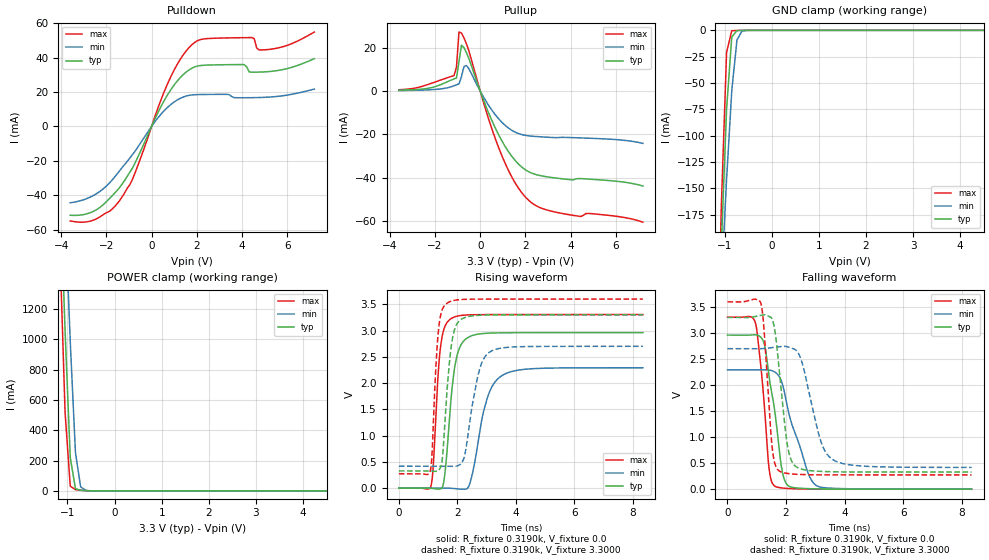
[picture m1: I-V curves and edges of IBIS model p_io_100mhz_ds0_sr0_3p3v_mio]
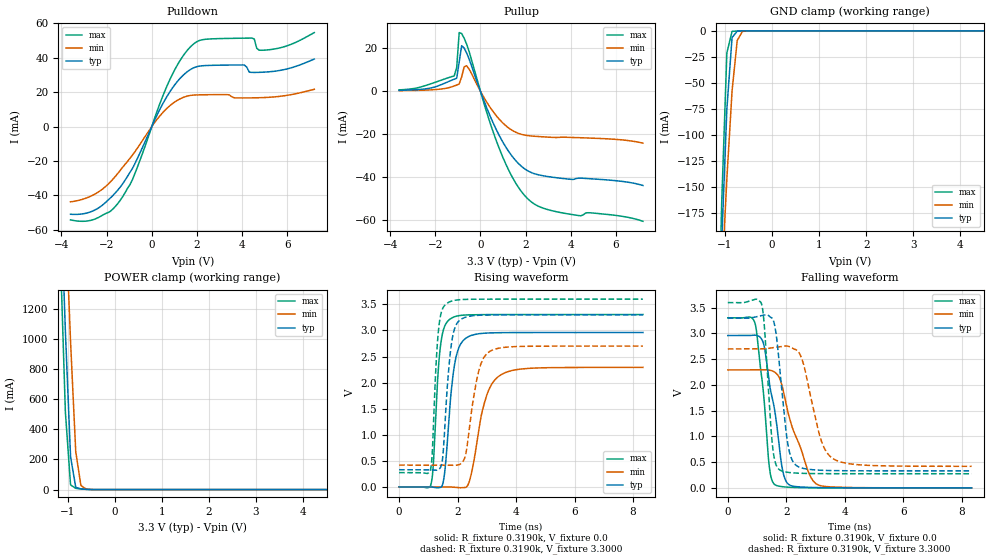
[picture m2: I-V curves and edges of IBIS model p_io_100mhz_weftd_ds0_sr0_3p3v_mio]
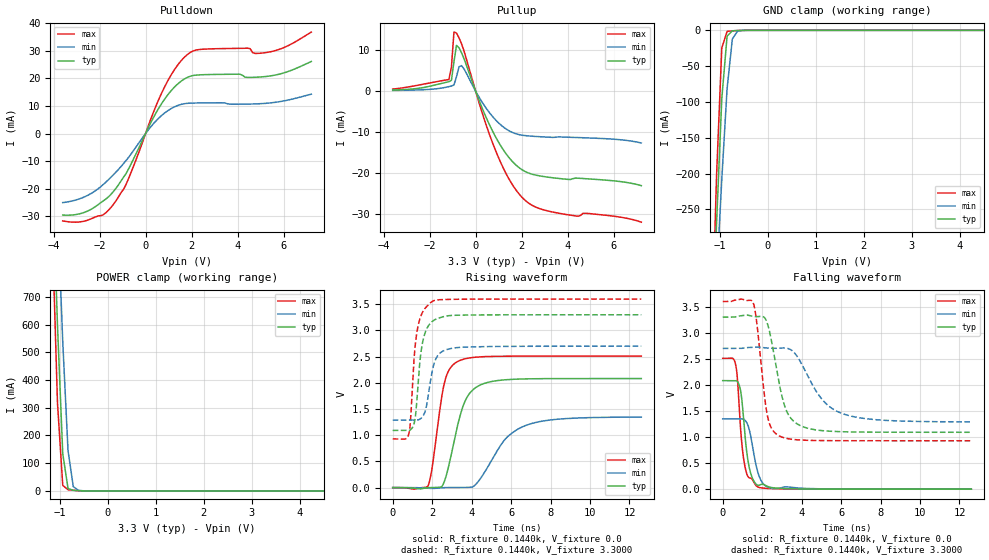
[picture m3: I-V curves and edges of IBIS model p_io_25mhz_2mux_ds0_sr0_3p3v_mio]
| IBIS file was generated by Viper version: 2025.12.22
[IBIS Ver]   6.0
[Comment Char]   |_char
[File Name]   c15x_c05x_24qfn.ibs
[File Rev]   1.0
[Date]   Fri Mar 13 19:24:16 2026
[Source]   NXP Viper 2025.12.22
[Notes]
[Disclaimer] IMPORTANT NOTICE
  This information is provided on an AS IS basis and without warranty.
  IN NO EVENT SHALL NXP BE LIABLE FOR INCIDENTAL OR CONSEQUENTIAL
  DAMAGES ARISING FROM USE OF THIS INFORMATION. THIS DISCLAIMER OF
  WARRANTY EXTENDS TO THE USER OF THE INFORMATION, AND TO THEIR CUSTOMERS
  OR USERS OF PRODUCTS  AND IS IN LIEU OF ALL WARRANTIES WHETHER EXPRESS,
  IMPLIED, OR STATUTORY, INCLUDING IMPLIED WARRANTIES OF MERCHANTABILITY
  OR FITNESS FOR PARTICULAR PURPOSE.
  NXP does not represent or warrant that the information furnished
  hereunder is free of infringement of any third party patents,
  copyrights, trade secrets, or other intellectual property rights.
  NXP does not represent or warrant that the information is free of
  defect, or that it meets any particular standard, requirements or need
  of the user of the infomation or their customers.
  NXP reserves the right to change the information in this file
  without notice.
   http://www.nxp.com
[Copyright]   (C) Copyright NXP 2004 - 2026, All Rights Reserved.
|   C15x_C05x_24QFN
[Component]   C15x_C05x_24QFN
[Manufacturer]   NXP
[Package]
| variable   typ   min   max
R_pkg   0.13896   0.12132   0.18535
L_pkg   1.804e-09   1.361e-09   2.436e-09
C_pkg   9.908e-14   8.894e-14   1.257e-13
[Pin] signal_name   model_name   R_pin   L_pin   C_pin
1   P1_9   a_ip_io_3v_3p3v   0.13781   1.901e-09 9.517e-14
2   P1_29   a_ip_io_3v_3p3v   0.12423   1.605e-09 9.039e-14
3   P1_30   a_ip_io_3v_3p3v   0.12132   1.528e-09 9.059e-14
4   P1_31   a_ip_io_3v_3p3v   0.13072   1.361e-09 1.032e-13
5   VDD   POWER   NA   NA   NA
6   P2_2   a_ip_io_3v_3p3v   0.14812   1.699e-09 1.013e-13
7   P2_3   a_ip_io_3v_3p3v   0.13439   1.749e-09 9.377e-14
8   P2_7   a_ip_io_3v_3p3v   0.12467   1.656e-09 9.088e-14
9   P2_12   a_ip_io_3v_3p3v   0.1273   1.509e-09 9.647e-14
10   P2_13   a_ip_io_3v_3p3v   0.13519   1.740e-09 1.000e-13
11   P2_16   a_ip_io_3v_3p3v   0.15539   1.988e-09 1.160e-13
12   P2_17   a_ip_io_3v_3p3v   0.18535   2.436e-09 1.257e-13
13   P3_29   a_ip_io_3v_3p3v   0.16284   2.122e-09 1.068e-13
14   P3_11   a_ip_io_3v_3p3v   0.14778   1.938e-09 1.010e-13
15   P3_10   a_ip_io_3v_3p3v   0.13217   1.797e-09 9.404e-14
16   P3_9   a_ip_io_3v_3p3v   0.12395   1.693e-09 9.041e-14
17   P3_8   a_ip_io_3v_3p3v   0.13055   1.797e-09 9.541e-14
18   P3_1   a_ip_io_3v_3p3v   0.15092   2.075e-09 1.056e-13
19   P3_0   a_ip_io_3v_3p3v   0.15252   1.996e-09 1.057e-13
20   P0_0   a_ip_io_3v_3p3v   0.12722   1.665e-09 9.034e-14
21   P0_1   a_ip_io_3v_3p3v   0.12378   1.709e-09 8.894e-14
22   P0_2   a_ip_io_3v_3p3v   0.13159   1.755e-09 9.620e-14
23   P0_3   a_ip_io_3v_3p3v   0.15143   1.961e-09 1.051e-13
24   P1_8   a_ip_io_3v_3p3v   0.13691   1.806e-09 9.582e-14
25   VSS   GND   NA   NA   NA
[Pin Mapping]   pulldown_ref   pullup_ref
1   VSS   VDD
2   VSS   VDD
3   VSS   VDD
4   VSS   VDD
5   NC   VDD
6   VSS   VDD
7   VSS   VDD
8   VSS   VDD
9   VSS   VDD
10   VSS   VDD
11   VSS   VDD
12   VSS   VDD
13   VSS   VDD
14   VSS   VDD
15   VSS   VDD
16   VSS   VDD
17   VSS   VDD
18   VSS   VDD
19   VSS   VDD
20   VSS   VDD
21   VSS   VDD
22   VSS   VDD
23   VSS   VDD
24   VSS   VDD
25   VSS   NC
|*   Model Selector   *
[Model Selector] a_ip_io_3v_3p3v
p_io_25mhz_ds0_sr0_3p3v_mio   dse=0 sre=0 25mhz
p_io_25mhz_ds0_sr1_3p3v_mio   dse=0 sre=1 25mhz
p_io_25mhz_ds1_sr0_3p3v_mio   dse=1 sre=0 25mhz
p_io_25mhz_ds1_sr1_3p3v_mio   dse=1 sre=1 25mhz
p_io_25mhz_r40_ds0_sr0_3p3v_mio   dse=0 sre=0 25mhz_r40
p_io_25mhz_r40_ds0_sr1_3p3v_mio   dse=0 sre=1 25mhz_r40
p_io_25mhz_r40_ds1_sr0_3p3v_mio   dse=1 sre=0 25mhz_r40
p_io_25mhz_r40_ds1_sr1_3p3v_mio   dse=1 sre=1 25mhz_r40
p_io_50mhz_ds0_sr0_3p3v_mio   dse=0 sre=0 50mhz
p_io_50mhz_ds0_sr1_3p3v_mio   dse=0 sre=1 50mhz
p_io_50mhz_ds1_sr0_3p3v_mio   dse=1 sre=0 50mhz
p_io_50mhz_ds1_sr1_3p3v_mio   dse=1 sre=1 50mhz
p_io_25mhz_cap_ds0_sr0_3p3v_mio   dse=0 sre=0 25mhz_cap
p_io_25mhz_cap_ds0_sr1_3p3v_mio   dse=0 sre=1 25mhz_cap
p_io_25mhz_cap_ds1_sr0_3p3v_mio   dse=1 sre=0 25mhz_cap
p_io_25mhz_cap_ds1_sr1_3p3v_mio   dse=1 sre=1 25mhz_cap
p_io_25mhz_2mux_ds0_sr0_3p3v_mio   dse=0 sre=0 25mhz_2mux
p_io_25mhz_2mux_ds0_sr1_3p3v_mio   dse=0 sre=1 25mhz_2mux
p_io_25mhz_2mux_ds1_sr0_3p3v_mio   dse=1 sre=0 25mhz_2mux
p_io_25mhz_2mux_ds1_sr1_3p3v_mio   dse=1 sre=1 25mhz_2mux
p_io_100mhz_ds0_sr0_3p3v_mio   dse=0 sre=0 100mhz
p_io_100mhz_ds0_sr1_3p3v_mio   dse=0 sre=1 100mhz
p_io_100mhz_ds1_sr0_3p3v_mio   dse=1 sre=0 100mhz
p_io_100mhz_ds1_sr1_3p3v_mio   dse=1 sre=1 100mhz
p_io_100mhz_weftd_ds0_sr0_3p3v_mio   dse=0 sre=0 100mhz
p_io_100mhz_weftd_ds0_sr1_3p3v_mio   dse=0 sre=1 100mhz
p_io_100mhz_weftd_ds1_sr0_3p3v_mio   dse=1 sre=0 100mhz
p_io_100mhz_weftd_ds1_sr1_3p3v_mio   dse=1 sre=1 100mhz
p_io_i2c_ds00_ds10_sr0_3p3v_mio   dse0=0 dse1=0 sre=0 i2c
p_io_i2c_ds00_ds10_sr1_3p3v_mio   dse0=0 dse1=0 sre=1 i2c
p_io_i2c_ds00_ds11_sr0_3p3v_mio   dse0=0 dse1=1 sre=0 i2c
p_io_i2c_ds00_ds11_sr1_3p3v_mio   dse0=0 dse1=1 sre=1 i2c
p_io_i2c_ds01_ds10_sr0_3p3v_mio   dse0=1 dse1=0 sre=0 i2c
p_io_i2c_ds01_ds10_sr1_3p3v_mio   dse0=1 dse1=0 sre=1 i2c
p_io_i2c_ds01_ds11_sr0_3p3v_mio   dse0=1 dse1=1 sre=0 i2c
p_io_i2c_ds01_ds11_sr1_3p3v_mio   dse0=1 dse1=1 sre=1 i2c
p_io_i2c_i2c1_3p3v_mio   ipp_i2c_lv=1 i2c
p_io_i2cfmp_ds00_ds10_sr0_3p3v_mio   dse0=0 dse1=0 sre=0 i2cfmp
p_io_i2cfmp_ds00_ds10_sr1_3p3v_mio   dse0=0 dse1=0 sre=1 i2cfmp
p_io_i2cfmp_ds00_ds11_sr0_3p3v_mio   dse0=0 dse1=1 sre=0 i2cfmp
p_io_i2cfmp_ds00_ds11_sr1_3p3v_mio   dse0=0 dse1=1 sre=1 i2cfmp
p_io_i2cfmp_ds01_ds10_sr0_3p3v_mio   dse0=1 dse1=0 sre=0 i2cfmp
p_io_i2cfmp_ds01_ds10_sr1_3p3v_mio   dse0=1 dse1=0 sre=1 i2cfmp
p_io_i2cfmp_ds01_ds11_sr0_3p3v_mio   dse0=1 dse1=1 sre=0 i2cfmp
p_io_i2cfmp_ds01_ds11_sr1_3p3v_mio   dse0=1 dse1=1 sre=1 i2cfmp
p_io_i2cfmp_i2c1_3p3v_mio   ipp_i2c_lv=1 i2cfmp
p_io_rst_3p3v_mio   rst
p_io_rst_rx1p8v_3p3v_mio   rst
p_io_aon_3p3v_mio   rst
| End [Component] C15x_C05x_24QFN
| Models and submodels in the file (49): p_io_100mhz_ds0_sr0_3p3v_mio (I/O), p_io_100mhz_ds0_sr1_3p3v_mio (I/O), p_io_100mhz_ds1_sr0_3p3v_mio (I/O), p_io_100mhz_ds1_sr1_3p3v_mio (I/O), p_io_100mhz_weftd_ds0_sr0_3p3v_mio (I/O), p_io_100mhz_weftd_ds0_sr1_3p3v_mio (I/O), p_io_100mhz_weftd_ds1_sr0_3p3v_mio (I/O), p_io_100mhz_weftd_ds1_sr1_3p3v_mio (I/O), p_io_25mhz_2mux_ds0_sr0_3p3v_mio (I/O), p_io_25mhz_2mux_ds0_sr1_3p3v_mio (I/O), p_io_25mhz_2mux_ds1_sr0_3p3v_mio (I/O), p_io_25mhz_2mux_ds1_sr1_3p3v_mio (I/O), p_io_25mhz_cap_ds0_sr0_3p3v_mio (I/O), p_io_25mhz_cap_ds0_sr1_3p3v_mio (I/O), p_io_25mhz_cap_ds1_sr0_3p3v_mio (I/O), p_io_25mhz_cap_ds1_sr1_3p3v_mio (I/O), p_io_25mhz_ds0_sr0_3p3v_mio (I/O), p_io_25mhz_ds0_sr1_3p3v_mio (I/O), p_io_25mhz_ds1_sr0_3p3v_mio (I/O), p_io_25mhz_ds1_sr1_3p3v_mio (I/O), p_io_25mhz_r40_ds0_sr0_3p3v_mio (I/O), p_io_25mhz_r40_ds0_sr1_3p3v_mio (I/O), p_io_25mhz_r40_ds1_sr0_3p3v_mio (I/O), p_io_25mhz_r40_ds1_sr1_3p3v_mio (I/O), p_io_50mhz_ds0_sr0_3p3v_mio (I/O), p_io_50mhz_ds0_sr1_3p3v_mio (I/O), p_io_50mhz_ds1_sr0_3p3v_mio (I/O), p_io_50mhz_ds1_sr1_3p3v_mio (I/O), p_io_aon_3p3v_mio (I/O), p_io_i2c_ds00_ds10_sr0_3p3v_mio (I/O), p_io_i2c_ds00_ds10_sr1_3p3v_mio (I/O), p_io_i2c_ds00_ds11_sr0_3p3v_mio (I/O), p_io_i2c_ds00_ds11_sr1_3p3v_mio (I/O), p_io_i2c_ds01_ds10_sr0_3p3v_mio (I/O), p_io_i2c_ds01_ds10_sr1_3p3v_mio (I/O), p_io_i2c_ds01_ds11_sr0_3p3v_mio (I/O), p_io_i2c_ds01_ds11_sr1_3p3v_mio (I/O), p_io_i2c_i2c1_3p3v_mio (I/O), p_io_i2cfmp_ds00_ds10_sr0_3p3v_mio (I/O), p_io_i2cfmp_ds00_ds10_sr1_3p3v_mio (I/O), p_io_i2cfmp_ds00_ds11_sr0_3p3v_mio (I/O), p_io_i2cfmp_ds00_ds11_sr1_3p3v_mio (I/O), p_io_i2cfmp_ds01_ds10_sr0_3p3v_mio (I/O), p_io_i2cfmp_ds01_ds10_sr1_3p3v_mio (I/O), p_io_i2cfmp_ds01_ds11_sr0_3p3v_mio (I/O), p_io_i2cfmp_ds01_ds11_sr1_3p3v_mio (I/O), p_io_i2cfmp_i2c1_3p3v_mio (I/O), p_io_rst_3p3v_mio (I/O), p_io_rst_rx1p8v_3p3v_mio (I/O)
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[Model] p_io_100mhz_ds0_sr0_3p3v_mio
|   Model p_io_100mhz_ds0_sr0_3p3v_mio
| This model was characterised for following simulation conditions:
| External (pad) voltage:
|   - Typ: 3.3V,   - Min: 2.7V,   - Max: 3.6V
| Library cells for typ/min/max conditions are connected as defined below:
|  pad - External Pad
|  ipp_do_lv - Core Input
|  ipp_obe_lv - Output Buffer Enable
|  IOGC - NC
|  REFH3V3 - REFH3V3
|  REFL3V3 - REFL3V3
|  ZI - NC
|  abut_ncal_vddio[1] - vddio
|  abut_ncal_vddio[2] - vddio
|  abut_ncal_vddio[3] - vssio
|  abut_ncal_vddio[4] - vddio
|  abut_ncal_vddio[5] - vddio
|  abut_ncal_vddio[6] - vssio
|  abut_pcal_vddio[1] - vssio
|  abut_pcal_vddio[2] - vssio
|  abut_pcal_vddio[3] - vddio
|  abut_pcal_vddio[4] - vssio
|  abut_pcal_vddio[5] - vssio
|  abut_pcal_vddio[6] - vddio
|  ipp_do_1p8v - ipp_do_1p8v
|  ipp_dse_lv - 0
|  ipp_eftd_lv - NC
|  ipp_ina_mux_vddio - NC
|  ipp_ina_mux_vddio[0] - NC
|  ipp_ina_mux_vddio[1] - NC
|  ipp_ina_r0_vddio - NC
|  ipp_ina_r0a_vddio - NC
|  ipp_ina_r0b_vddio - NC
|  ipp_ina_r0c_vddio - NC
|  ipp_ina_r0d_vddio - NC
|  ipp_ina_r0e_vddio - NC
|  ipp_ina_r0f_vddio - NC
|  ipp_ina_r300_vddio - NC
|  ipp_ina_r300a_vddio - NC
|  ipp_ina_r300b_vddio - NC
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Model_type I/O
Polarity   Non-Inverting
Enable   Active-High
Vinl =   0.9900V
Vinh =   2.3100V
Vmeas =  1.6500V
Cref =   30.0000pF
Rref =   1.0000M
Vref =   3.3000V
C_comp   1.3235pF   1.2640pF   1.4076pF
|C_comp_pullup   0.6739pF   0.7056pF   0.6519pF
|C_comp_pulldown   0.5816pF   0.6344pF   0.5434pF
[Model Spec]
| variable   typ   min   max
Vinh   2.3100V   1.8900V   2.5200V
Vinl   0.9900V   0.8100V   1.0800V
[Temperature Range]   25.0000   0.1250k   -40.0000
[Voltage Range]   3.3000V   2.7000V   3.6000V
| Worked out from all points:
|   slope of the pulldown table from 0 to 0.495 V, typ, clamps not added: 36.6 ohm
|   slope of the pullup table from 0 to 0.495 V, typ, clamps not added: 37.7 ohm
|   GND clamp passes 1 mA (typ) near -0.75 V on its own axis
|   POWER clamp passes 1 mA (typ) near -0.55 V on its own axis
|   rising waveform, R_fixture 0.3190k, V_fixture 0.0: 20-80 % time 299ps typ, 517ps min, 214ps max; typ from 0 V to 2.96 V
|   rising waveform, R_fixture 0.3190k, V_fixture 3.3000: 20-80 % time 255ps typ, 423ps min, 184ps max; typ from 0.328 V to 3.3 V
|   falling waveform, R_fixture 0.3190k, V_fixture 0.0: 20-80 % time 427ps typ, 707ps min, 290ps max; typ from 2.96 V to 0 V
|   falling waveform, R_fixture 0.3190k, V_fixture 3.3000: 20-80 % time 330ps typ, 583ps min, 237ps max; typ from 3.3 V to 0.329 V
[Pulldown]
|Voltage   I(typ)   I(min)   I(max)
-3.6V     -51.52mA   -44.27mA   -54.81mA
-2.5V     -48.75mA   -39.51mA   -53.96mA
-1.4V     -35.12mA   -25.45mA   -42.73mA
-850mV    -24.27mA   -16.41mA   -30.84mA
800mV     20.29mA    12.16mA    27.43mA
1.35V     29.44mA    16.78mA    40.57mA
1.9V      34.5mA     18.39mA    48.67mA
4.1V      35.87mA    16.66mA    51.51mA
4.43V     31.5mA     16.69mA    51.59mA
4.65V     31.5mA     16.75mA    45.53mA
5.09V     31.75mA    16.96mA    44.55mA
7.2V      39.3mA     21.67mA    54.74mA
[Pullup]
|Voltage   I(typ)   I(min)   I(max)
-3.6V     391.8uA    234.9uA    605.7uA
-1.16V    5.604mA    2.419mA    7.14mA
-1.05V    6.055mA    2.871mA    11mA
-940mV    13.56mA    3.339mA    27.24mA
-830mV    21.15mA    6.685mA    26.82mA
-720mV    20.05mA    11.26mA    24.61mA
-610mV    17.74mA    11.81mA    21.86mA
820mV     -20.29mA   -12.86mA   -26.23mA
1.48V     -31.23mA   -18.63mA   -41.23mA
2.03V     -36.57mA   -20.53mA   -49.31mA
3.46V     -40.33mA   -21.49mA   -56.22mA
7.2V      -43.87mA   -24.17mA   -60.58mA
[GND_clamp]
|Voltage   I(typ)   I(min)   I(max)
-3.6V     -4.134A    -3.035A    -5.609A
-1.18V    -349.4mA   -343.6mA   -365.7mA
-1.07V    -202.9mA   -239.3mA   -165.2mA
-960mV    -74.83mA   -141.5mA   -21.03mA
-850mV    -6.389mA   -57.64mA   -383.3uA
-740mV    -222.1uA   -9.174mA   -124.1uA
-630mV    -55.93uA   -558.9uA   -58.07uA
7.2V      0A         0A         0A
[POWER_clamp]
|Voltage   I(typ)   I(min)   I(max)
-3.6V     24.54A     22.33A     26.93A
-1.16V    2.046A     2.721A     1.599A
-1.05V    1.052A     1.847A     514.4mA
-940mV    218.6mA    981.8mA    31.16mA
-830mV    15.1mA     252.4mA    8.462mA
-720mV    4.281mA    26.81mA    4.453mA
-610mV    1.717mA    3.626mA    1.66mA
7.2V      0A         0A         0A
[Ramp]
| variable   typ   min   max
dV/dt_r  1.7763/0.2988n   1.3750/0.5172n   1.9832/0.2140n
dV/dt_f  1.7829/0.3304n   1.3692/0.5829n   1.9962/0.2366n
R_load = 0.3190k
[Rising Waveform]
R_fixture= 0.3190k
V_fixture= 0.0
V_fixture_min= 0.0
V_fixture_max= 0.0
|time   V(typ)   V(min)   V(max)
0s        2.902nV    250nV      9.459nV
1.086ns   -976.7uV   -29.66uV   18.83mV
1.414ns   -15.5mV    651.1uV    2.638V
1.567ns   247.8mV    1.45mV     3.071V
1.766ns   1.596V     -2.144mV   3.22V
2.173ns   2.772V     -19.8mV    3.292V
2.455ns   2.894V     144.2mV    3.3V
3.05ns    2.95V      1.761V     3.304V
3.542ns   2.957V     2.149V     3.305V
8.34ns    2.961V     2.292V     3.305V
[Rising Waveform]
R_fixture= 0.3190k
V_fixture= 3.3000
V_fixture_min= 2.7000
V_fixture_max= 3.6000
|time   V(typ)   V(min)   V(max)
0s        328.4mV    417.4mV    273mV
1.073ns   327.9mV    417.3mV    324.4mV
1.356ns   339mV      417.7mV    3.019V
1.484ns   549.3mV    418.3mV    3.402V
1.64ns    1.817V     417.6mV    3.518V
1.974ns   3.118V     421.1mV    3.583V
2.25ns    3.247V     626.3mV    3.595V
2.767ns   3.292V     2.277V     3.599V
3.119ns   3.297V     2.597V     3.6V
8.34ns    3.3V       2.7V       3.6V
[Falling Waveform]
R_fixture= 0.3190k
V_fixture= 0.0
V_fixture_min= 0.0
V_fixture_max= 0.0
|time   V(typ)   V(min)   V(max)
0s        2.961V     2.292V     3.305V
954.1ps   2.967V     2.291V     3.197V
1.243ns   2.815V     2.294V     1.731V
1.42ns    2.166V     2.29V      403.1mV
1.604ns   1.548V     2.256V     63.43mV
1.828ns   486.1mV    2.1V       25.24mV
1.982ns   134.6mV    1.766V     16.49mV
2.726ns   10.64mV    351.6mV    2.556mV
3.05ns    5.57mV     66.35mV    1.221mV
8.34ns    83.62uV    191.3uV    53.48uV
[Falling Waveform]
R_fixture= 0.3190k
V_fixture= 3.3000
V_fixture_min= 2.7000
V_fixture_max= 3.6000
|time   V(typ)   V(min)   V(max)
0s        3.3V       2.7V       3.6V
1.141ns   3.342V     2.699V     3.572V
1.245ns   3.351V     2.703V     3.102V
1.533ns   3.259V     2.721V     770.1mV
1.769ns   2.279V     2.737V     349.2mV
2.06ns    805.8mV    2.736V     300.7mV
2.402ns   411.8mV    2.631V     284mV
3.171ns   341.9mV    951.9mV    274.9mV
3.588ns   334.4mV    572.4mV    273.9mV
8.34ns    328.6mV    418.1mV    273.1mV
[Model] p_io_100mhz_weftd_ds0_sr0_3p3v_mio
|   Model p_io_100mhz_weftd_ds0_sr0_3p3v_mio
| This model was characterised for following simulation conditions:
| External (pad) voltage:
|   - Typ: 3.3V,   - Min: 2.7V,   - Max: 3.6V
| Library cells for typ/min/max conditions are connected as defined below:
|  pad - External Pad
|  ipp_do_lv - Core Input
|  ipp_obe_lv - Output Buffer Enable
|  IOGC - NC
|  REFH3V3 - REFH3V3
|  REFL3V3 - REFL3V3
|  ZI - NC
|  abut_ncal_vddio[1] - vddio
|  abut_ncal_vddio[2] - vddio
|  abut_ncal_vddio[3] - vssio
|  abut_ncal_vddio[4] - vddio
|  abut_ncal_vddio[5] - vddio
|  abut_ncal_vddio[6] - vssio
|  abut_pcal_vddio[1] - vssio
|  abut_pcal_vddio[2] - vssio
|  abut_pcal_vddio[3] - vddio
|  abut_pcal_vddio[4] - vssio
|  abut_pcal_vddio[5] - vssio
|  abut_pcal_vddio[6] - vddio
|  ipp_do_1p8v - ipp_do_1p8v
|  ipp_dse_lv - 0
|  ipp_eftd_lv - NC
|  ipp_ina_mux_vddio - NC
|  ipp_ina_mux_vddio[0] - NC
|  ipp_ina_mux_vddio[1] - NC
|  ipp_ina_r0_vddio - NC
|  ipp_ina_r0a_vddio - NC
|  ipp_ina_r0b_vddio - NC
|  ipp_ina_r0c_vddio - NC
|  ipp_ina_r0d_vddio - NC
|  ipp_ina_r0e_vddio - NC
|  ipp_ina_r0f_vddio - NC
|  ipp_ina_r300_vddio - NC
|  ipp_ina_r300a_vddio - NC
|  ipp_ina_r300b_vddio - NC
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Model_type I/O
Polarity   Non-Inverting
Enable   Active-High
Vinl =   0.9900V
Vinh =   2.3100V
Vmeas =  1.6500V
Cref =   30.0000pF
Rref =   1.0000M
Vref =   3.3000V
C_comp   1.3824pF   1.3233pF   1.4661pF
|C_comp_pullup   0.6923pF   0.7238pF   0.6706pF
|C_comp_pulldown   0.6090pF   0.6618pF   0.5704pF
[Model Spec]
| variable   typ   min   max
Vinh   2.3100V   1.8900V   2.5200V
Vinl   0.9900V   0.8100V   1.0800V
[Temperature Range]   25.0000   0.1250k   -40.0000
[Voltage Range]   3.3000V   2.7000V   3.6000V
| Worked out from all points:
|   slope of the pulldown table from 0 to 0.495 V, typ, clamps not added: 36.8 ohm
|   slope of the pullup table from 0 to 0.495 V, typ, clamps not added: 37.8 ohm
|   GND clamp passes 1 mA (typ) near -0.75 V on its own axis
|   POWER clamp passes 1 mA (typ) near -0.55 V on its own axis
|   rising waveform, R_fixture 0.3190k, V_fixture 0.0: 20-80 % time 291ps typ, 502ps min, 208ps max; typ from 0 V to 2.96 V
|   rising waveform, R_fixture 0.3190k, V_fixture 3.3000: 20-80 % time 241ps typ, 386ps min, 177ps max; typ from 0.33 V to 3.3 V
|   falling waveform, R_fixture 0.3190k, V_fixture 0.0: 20-80 % time 457ps typ, 746ps min, 320ps max; typ from 2.96 V to 0 V
|   falling waveform, R_fixture 0.3190k, V_fixture 3.3000: 20-80 % time 322ps typ, 565ps min, 230ps max; typ from 3.3 V to 0.33 V
[Pulldown]
|Voltage   I(typ)   I(min)   I(max)
-3.6V     -50.99mA   -43.76mA   -54.26mA
-2.5V     -48.39mA   -39.11mA   -53.69mA
-1.4V     -35.22mA   -25.46mA   -42.92mA
-850mV    -24.19mA   -16.4mA    -30.69mA
800mV     20.23mA    12.14mA    27.32mA
1.35V     29.37mA    16.76mA    40.44mA
1.9V      34.45mA    18.38mA    48.57mA
4.1V      35.83mA    16.68mA    51.45mA
4.43V     31.54mA    16.72mA    51.52mA
4.65V     31.54mA    16.77mA    45.56mA
5.09V     31.78mA    16.98mA    44.58mA
7.2V      39.32mA    21.7mA     54.71mA
[Pullup]
|Voltage   I(typ)   I(min)   I(max)
-3.6V     392.3uA    235.2uA    607.2uA
-1.16V    5.571mA    2.41mA     7.094mA
-1.05V    6.017mA    2.857mA    10.99mA
-940mV    13.55mA    3.321mA    27.21mA
-830mV    21.12mA    6.673mA    26.77mA
-720mV    20.02mA    11.25mA    24.57mA
-610mV    17.72mA    11.8mA     21.82mA
820mV     -20.27mA   -12.85mA   -26.19mA
1.48V     -31.2mA    -18.62mA   -41.17mA
2.03V     -36.53mA   -20.52mA   -49.25mA
3.46V     -40.29mA   -21.47mA   -56.15mA
7.2V      -43.77mA   -24.12mA   -60.4mA
[GND_clamp]
|Voltage   I(typ)   I(min)   I(max)
-3.6V     -4.179A    -3.084A    -5.65A
-1.18V    -350.3mA   -344.8mA   -366.5mA
-1.07V    -203.5mA   -240.3mA   -165.6mA
-960mV    -75.17mA   -142.1mA   -21.27mA
-850mV    -6.53mA    -58.02mA   -538.4uA
-740mV    -289.9uA   -9.332mA   -209.1uA
-630mV    -85.04uA   -601.4uA   -92.54uA
-300mV    -199.1nA   -1.25uA    -48.79nA
7.2V      0A         0A         0A
[POWER_clamp]
|Voltage   I(typ)   I(min)   I(max)
-3.6V     24.55A     22.33A     26.93A
-1.16V    2.047A     2.721A     1.599A
-1.05V    1.052A     1.848A     514.6mA
-940mV    218.8mA    982.2mA    31.26mA
-830mV    15.16mA    252.6mA    8.517mA
-720mV    4.307mA    26.88mA    4.483mA
-610mV    1.728mA    3.641mA    1.672mA
7.2V      0A         0A         0A
[Ramp]
| variable   typ   min   max
dV/dt_r  1.7760/0.2909n   1.3748/0.5021n   1.9829/0.2081n
dV/dt_f  1.7821/0.3218n   1.3686/0.5645n   1.9953/0.2303n
R_load = 0.3190k
[Rising Waveform]
R_fixture= 0.3190k
V_fixture= 0.0
V_fixture_min= 0.0
V_fixture_max= 0.0
|time   V(typ)   V(min)   V(max)
0s        3.011nV    251.5nV    9.8nV
1.08ns    -136.2uV   -133.7uV   31.45mV
1.403ns   -9.863mV   462.1uV    2.652V
1.554ns   257.9mV    1.193mV    3.075V
1.748ns   1.627V     -806.3uV   3.22V
2.152ns   2.779V     -14.57mV   3.291V
2.429ns   2.896V     158.7mV    3.299V
3.011ns   2.95V      1.78V      3.304V
3.48ns    2.957V     2.149V     3.304V
8.34ns    2.96V      2.291V     3.305V
[Rising Waveform]
R_fixture= 0.3190k
V_fixture= 3.3000
V_fixture_min= 2.7000
V_fixture_max= 3.6000
|time   V(typ)   V(min)   V(max)
0s        329.6mV    418.3mV    274.4mV
1.067ns   329.7mV    418.1mV    319.9mV
1.345ns   331.6mV    418.4mV    3V
1.492ns   570mV      419.1mV    3.423V
1.639ns   1.858V     418.6mV    3.521V
1.956ns   3.114V     416.5mV    3.582V
2.259ns   3.251V     582.3mV    3.595V
2.687ns   3.29V      2.14V      3.599V
3.085ns   3.297V     2.593V     3.599V
8.34ns    3.3V       2.7V       3.6V
[Falling Waveform]
R_fixture= 0.3190k
V_fixture= 0.0
V_fixture_min= 0.0
V_fixture_max= 0.0
|time   V(typ)   V(min)   V(max)
0s        2.96V      2.291V     3.305V
935.6ps   2.967V     2.29V      3.192V
1.225ns   2.8V       2.293V     1.823V
1.421ns   2.042V     2.288V     407.2mV
1.613ns   1.48V      2.246V     61.66mV
1.84ns    454.3mV    2.021V     24.44mV
2.002ns   121.3mV    1.613V     15.48mV
2.745ns   9.966mV    329.1mV    2.309mV
3.058ns   5.239mV    67.31mV    1.158mV
8.34ns    86.65uV    196.2uV    54.92uV
[Falling Waveform]
R_fixture= 0.3190k
V_fixture= 3.3000
V_fixture_min= 2.7000
V_fixture_max= 3.6000
|time   V(typ)   V(min)   V(max)
0s        3.3V       2.7V       3.6V
1.156ns   3.349V     2.7V       3.575V
1.258ns   3.363V     2.704V     3.099V
1.531ns   3.287V     2.723V     814.5mV
1.768ns   2.378V     2.741V     352.3mV
2.062ns   828.8mV    2.753V     301.6mV
2.398ns   415mV      2.657V     285.3mV
3.181ns   342.3mV    946.9mV    276.3mV
3.592ns   335.4mV    571.7mV    275.4mV
8.34ns    329.8mV    419mV      274.5mV
[Model] p_io_25mhz_2mux_ds0_sr0_3p3v_mio
|   Model p_io_25mhz_2mux_ds0_sr0_3p3v_mio
| This model was characterised for following simulation conditions:
| External (pad) voltage:
|   - Typ: 3.3V,   - Min: 2.7V,   - Max: 3.6V
| Library cells for typ/min/max conditions are connected as defined below:
|  pad - External Pad
|  ipp_do_lv - Core Input
|  ipp_obe_lv - Output Buffer Enable
|  IOGC - NC
|  REFH3V3 - REFH3V3
|  REFL3V3 - REFL3V3
|  ZI - NC
|  abut_ncal_vddio[1] - vddio
|  abut_ncal_vddio[2] - vddio
|  abut_ncal_vddio[3] - vssio
|  abut_ncal_vddio[4] - vddio
|  abut_ncal_vddio[5] - vddio
|  abut_ncal_vddio[6] - vssio
|  abut_pcal_vddio[1] - vssio
|  abut_pcal_vddio[2] - vssio
|  abut_pcal_vddio[3] - vddio
|  abut_pcal_vddio[4] - vssio
|  abut_pcal_vddio[5] - vssio
|  abut_pcal_vddio[6] - vddio
|  ipp_do_1p8v - ipp_do_1p8v
|  ipp_dse_lv - 0
|  ipp_eftd_lv - NC
|  ipp_ina_mux_vddio - NC
|  ipp_ina_mux_vddio[0] - NC
|  ipp_ina_mux_vddio[1] - NC
|  ipp_ina_r0_vddio - NC
|  ipp_ina_r0a_vddio - NC
|  ipp_ina_r0b_vddio - NC
|  ipp_ina_r0c_vddio - NC
|  ipp_ina_r0d_vddio - NC
|  ipp_ina_r0e_vddio - NC
|  ipp_ina_r0f_vddio - NC
|  ipp_ina_r300_vddio - NC
|  ipp_ina_r300a_vddio - NC
|  ipp_ina_r300b_vddio - NC
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Model_type I/O
Polarity   Non-Inverting
Enable   Active-High
Vinl =   0.9900V
Vinh =   2.3100V
Vmeas =  1.6500V
Cref =   30.0000pF
Rref =   1.0000M
Vref =   3.3000V
C_comp   1.2811pF   1.2303pF   1.3501pF
|C_comp_pullup   0.5369pF   0.5681pF   0.5156pF
|C_comp_pulldown   0.6705pF   0.7072pF   0.6414pF
[Model Spec]
| variable   typ   min   max
Vinh   2.3100V   1.8900V   2.5200V
Vinl   0.9900V   0.8100V   1.0800V
[Temperature Range]   25.0000   0.1250k   -40.0000
[Voltage Range]   3.3000V   2.7000V   3.6000V
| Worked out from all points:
|   slope of the pulldown table from 0 to 0.495 V, typ, clamps not added: 61.2 ohm
|   slope of the pullup table from 0 to 0.495 V, typ, clamps not added: 71.7 ohm
|   GND clamp passes 1 mA (typ) near -0.74 V on its own axis
|   POWER clamp passes 1 mA (typ) near -0.62 V on its own axis
|   rising waveform, R_fixture 0.1440k, V_fixture 0.0: 20-80 % time 844ps typ, 1.56ns min, 580ps max; typ from 0 V to 2.08 V
|   rising waveform, R_fixture 0.1440k, V_fixture 3.3000: 20-80 % time 369ps typ, 423ps min, 341ps max; typ from 1.09 V to 3.3 V
|   falling waveform, R_fixture 0.1440k, V_fixture 0.0: 20-80 % time 360ps typ, 440ps min, 328ps max; typ from 2.08 V to 0 V
|   falling waveform, R_fixture 0.1440k, V_fixture 3.3000: 20-80 % time 733ps typ, 1.47ns min, 471ps max; typ from 3.3 V to 1.09 V
[Pulldown]
|Voltage   I(typ)   I(min)   I(max)
-3.6V     -29.55mA   -25.02mA   -31.65mA
-2.5V     -28.03mA   -22.34mA   -31.35mA
-1.84V    -24.43mA   -18.49mA   -29.45mA
-1.4V     -21.05mA   -14.95mA   -25.71mA
-850mV    -14.55mA   -9.778mA   -18.51mA
800mV     12.15mA    7.264mA    16.45mA
1.35V     17.61mA    10.02mA    24.32mA
1.9V      20.65mA    11mA       29.17mA
4.43V     20.35mA    10.67mA    30.94mA
4.76V     20.4mA     10.74mA    29.03mA
5.31V     20.76mA    11.01mA    29.46mA
7.2V      26.12mA    14.27mA    36.77mA
[Pullup]
|Voltage   I(typ)   I(min)   I(max)
-3.6V     250.7uA    138.3uA    483.6uA
-1.16V    2.271mA    1.069mA    2.801mA
-1.05V    2.603mA    1.213mA    5.776mA
-940mV    7.093mA    1.465mA    14.38mA
-830mV    11.13mA    3.481mA    14.15mA
-720mV    10.55mA    5.904mA    12.99mA
-610mV    9.336mA    6.198mA    11.54mA
820mV     -10.68mA   -6.749mA   -13.84mA
1.48V     -16.43mA   -9.783mA   -21.75mA
2.03V     -19.25mA   -10.79mA   -26.01mA
3.35V     -21.16mA   -11.31mA   -29.53mA
7.2V      -23.09mA   -12.68mA   -32mA
[GND_clamp]
|Voltage   I(typ)   I(min)   I(max)
-3.6V     -5.309A    -4.128A    -6.876A
-1.18V    -466mA     -495.4mA   -458.9mA
-1.07V    -271.1mA   -348.5mA   -204.6mA
-960mV    -95.65mA   -208mA     -24.74mA
-850mV    -8.096mA   -81.85mA   -1.474mA
-740mV    -719.7uA   -12.14mA   -719.4uA
-630mV    -272.5uA   -923.5uA   -301.7uA
-300mV    -385.6nA   -2.502uA   -74.93nA
7.2V      0A         0A         0A
[POWER_clamp]
|Voltage   I(typ)   I(min)   I(max)
-3.6V     14.48A     12.95A     16.35A
-1.16V    1.177A     1.535A     951.2mA
-1.05V    598.4mA    1.032A     318mA
-940mV    134.2mA    537.3mA    20.02mA
-830mV    8.708mA    145.4mA    4.242mA
-720mV    2.127mA    15.38mA    2.218mA
-610mV    847.4uA    1.853mA    834.1uA
7.2V      0A         0A         0A
[Ramp]
| variable   typ   min   max
dV/dt_r  1.2492/0.8441n   0.8078/1.5632n   1.5061/0.5798n
dV/dt_f  1.3253/0.7333n   0.8457/1.4717n   1.6029/0.4715n
R_load = 0.1440k
[Rising Waveform]
R_fixture= 0.1440k
V_fixture= 0.0
V_fixture_min= 0.0
V_fixture_max= 0.0
|time   V(typ)   V(min)   V(max)
0s        4.603nV    154.1nV    15.8nV
1.784ns   -2.583mV   -13.13mV   27.47mV
1.988ns   647.7uV    -16.58mV   357mV
2.603ns   102.3mV    -809.1uV   1.973V
3.264ns   1.149V     1.101mV    2.402V
3.824ns   1.76V      3.183mV    2.471V
4.799ns   2.007V     380.9mV    2.503V
5.757ns   2.06V      947.3mV    2.509V
6.827ns   2.076V     1.198V     2.51V
12.6ns    2.082V     1.346V     2.51V
[Rising Waveform]
R_fixture= 0.1440k
V_fixture= 3.3000
V_fixture_min= 2.7000
V_fixture_max= 3.6000
|time   V(typ)   V(min)   V(max)
0s        1.091V     1.288V     928.6mV
808.6ps   1.091V     1.288V     1.015V
902.3ps   1.103V     1.288V     1.283V
1.055ns   1.19V      1.289V     2.311V
1.225ns   1.663V     1.289V     2.964V
1.489ns   2.722V     1.344V     3.331V
2.015ns   3.175V     2.246V     3.558V
2.365ns   3.241V     2.558V     3.587V
3.24ns    3.291V     2.672V     3.596V
12.6ns    3.3V       2.7V       3.6V
[Falling Waveform]
R_fixture= 0.1440k
V_fixture= 0.0
V_fixture_min= 0.0
V_fixture_max= 0.0
|time   V(typ)   V(min)   V(max)
0s        2.082V     1.348V     2.51V
616.7ps   2.083V     1.348V     2.443V
726.5ps   2.071V     1.348V     2.202V
836.5ps   1.995V     1.348V     1.571V
981.1ps   1.676V     1.349V     829.3mV
1.162ns   900.2mV    1.309V     374mV
1.408ns   317.4mV    1.038V     214.6mV
1.786ns   75.23mV    316.7mV    41.7mV
2.634ns   22.76mV    12.15mV    7.932mV
12.6ns    198.7nV    13.86uV    45.49nV
[Falling Waveform]
R_fixture= 0.1440k
V_fixture= 3.3000
V_fixture_min= 2.7000
V_fixture_max= 3.6000
|time   V(typ)   V(min)   V(max)
0s        3.3V       2.7V       3.6V
1.546ns   3.315V     2.723V     3.575V
1.72ns    3.308V     2.726V     3.217V
2.266ns   3.176V     2.707V     1.408V
2.856ns   2.037V     2.706V     1.023V
3.207ns   1.524V     2.706V     975.6mV
3.648ns   1.287V     2.61V      950.5mV
5.01ns    1.124V     1.735V     932mV
6.047ns   1.102V     1.452V     929.7mV
12.6ns    1.091V     1.29V      928.6mV
